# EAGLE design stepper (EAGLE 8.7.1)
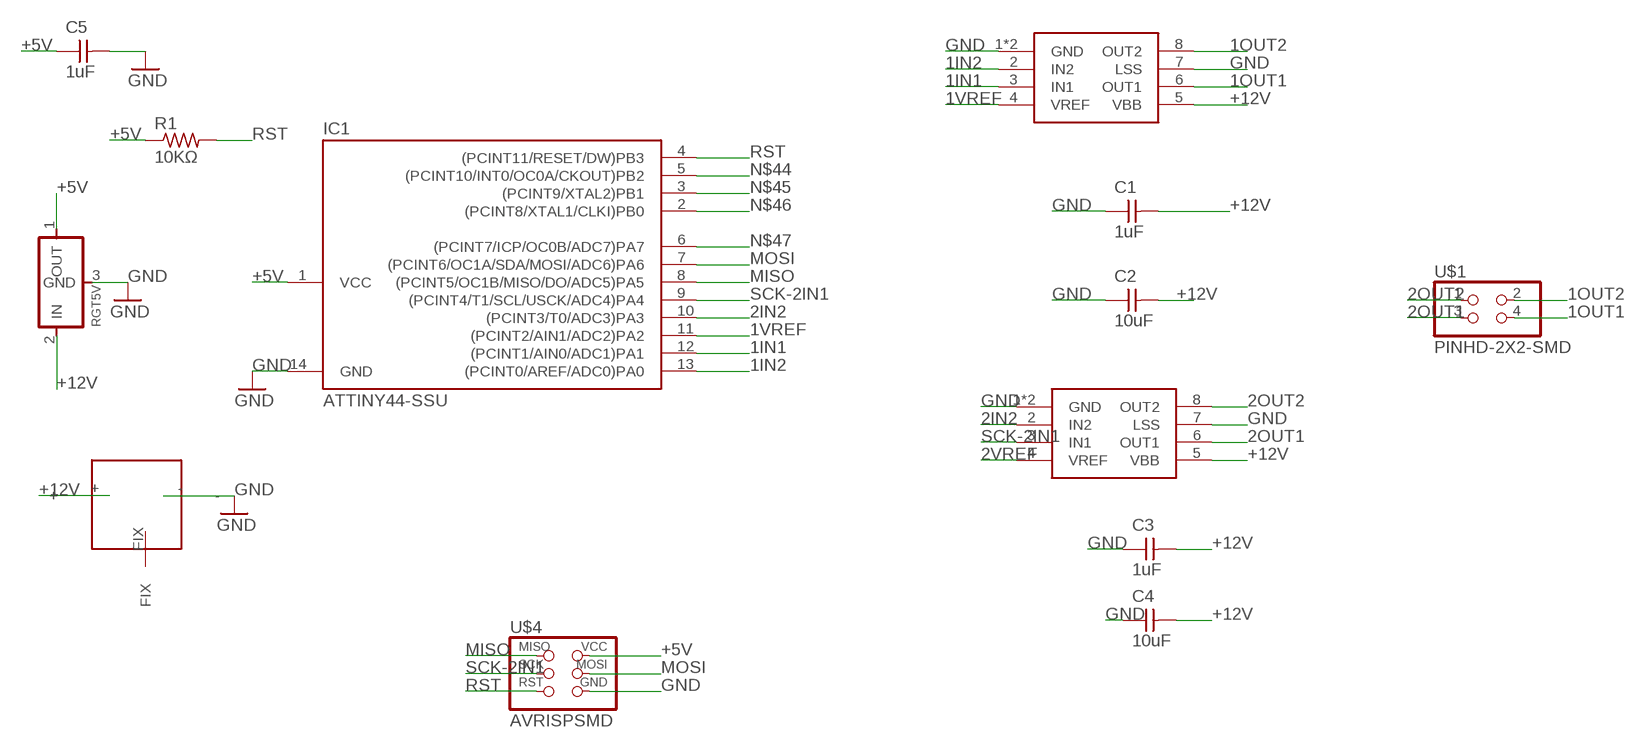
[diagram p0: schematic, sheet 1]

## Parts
C1  1uF  CAP-UNPOLARIZEDFAB  [C1206FAB]
C2  10uF  CAP-UNPOLARIZEDFAB  [C1206FAB]
C3  1uF  CAP-UNPOLARIZEDFAB  [C1206FAB]
C4  10uF  CAP-UNPOLARIZEDFAB  [C1206FAB]
C5  1uF  CAP-UNPOLARIZEDFAB  [C1206FAB]
DCJACK1  AKIZUKI_DCJACK  [AKIZUKI_DCJACK]
IC1  ATTINY44-SSU  [SOIC14]
R1  10KΩ  RES-US1206FAB  [R1206FAB]
RGT5V  REGULATORSOT23  [SOT23]
U$1  PINHD-2X2-SMD  [2X02SMD]
U$2  A4953-H-BRIDGE-MOTOR-DRIVER-PAD  [SOIC8_PAD]
U$3  A4953-H-BRIDGE-MOTOR-DRIVER-PAD  [SOIC8_PAD]
U$4  AVRISPSMD  [2X03SMD]

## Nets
1IN1: IC1.12((PCINT1/AIN0/ADC1)PA1) U$3.3(IN1)
1IN2: IC1.13((PCINT0/AREF/ADC0)PA0) U$3.2(IN2)
1OUT1: U$1.4 U$3.6(OUT1)
1OUT2: U$1.2 U$3.8(OUT2)
1VREF: IC1.11((PCINT2/AIN1/ADC2)PA2) U$3.4(VREF)
2IN2: IC1.10((PCINT3/T0/ADC3)PA3) U$2.2(IN2)
2OUT1: U$1.3 U$2.6(OUT1)
2OUT2: U$1.1 U$2.8(OUT2)
2VREF: U$2.4(VREF)
+5V: C5.1 IC1.1(VCC) R1.1 RGT5V.1(OUT) U$4.2(VCC)
+12V: C1.2 C2.2 C3.2 C4.2 DCJACK1.+ RGT5V.2(IN) U$2.5(VBB) U$3.5(VBB)
GND: C1.1 C2.1 C3.1 C4.1 C5.2 DCJACK1.- IC1.14(GND) RGT5V.3(GND) U$2.1(GND) U$2.7(LSS) U$2.GND U$3.1(GND) U$3.7(LSS) U$3.GND U$4.6(GND)
MISO: IC1.8((PCINT5/OC1B/MISO/DO/ADC5)PA5) U$4.1(MISO)
MOSI: IC1.7((PCINT6/OC1A/SDA/MOSI/ADC6)PA6) U$4.4(MOSI)
N$44: IC1.5((PCINT10/INT0/OC0A/CKOUT)PB2)
N$45: IC1.3((PCINT9/XTAL2)PB1)
N$46: IC1.2((PCINT8/XTAL1/CLKI)PB0)
N$47: IC1.6((PCINT7/ICP/OC0B/ADC7)PA7)
RST: IC1.4((PCINT11/RESET/DW)PB3) R1.2 U$4.5(RST)
SCK-2IN1: IC1.9((PCINT4/T1/SCL/USCK/ADC4)PA4) U$2.3(IN1) U$4.3(SCK)
Unconnected: DCJACK1.FIX

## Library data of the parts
C1-C5 = fab:CAP-UNPOLARIZED
DCJACK1 = doyo:AKIZUKI_DCJACK
IC1 = fab:ATTINY44
R1 = HelloKamakura:RES-US: Resistor (US Symbol)
RGT5V = fab:REGULATOR
U$1 = fab:PINHD-2X2-SMD
U$2 U$3 = fab:A4953-H-BRIDGE-MOTOR-DRIVER-PAD
U$4 = HelloKamakura:AVRISP

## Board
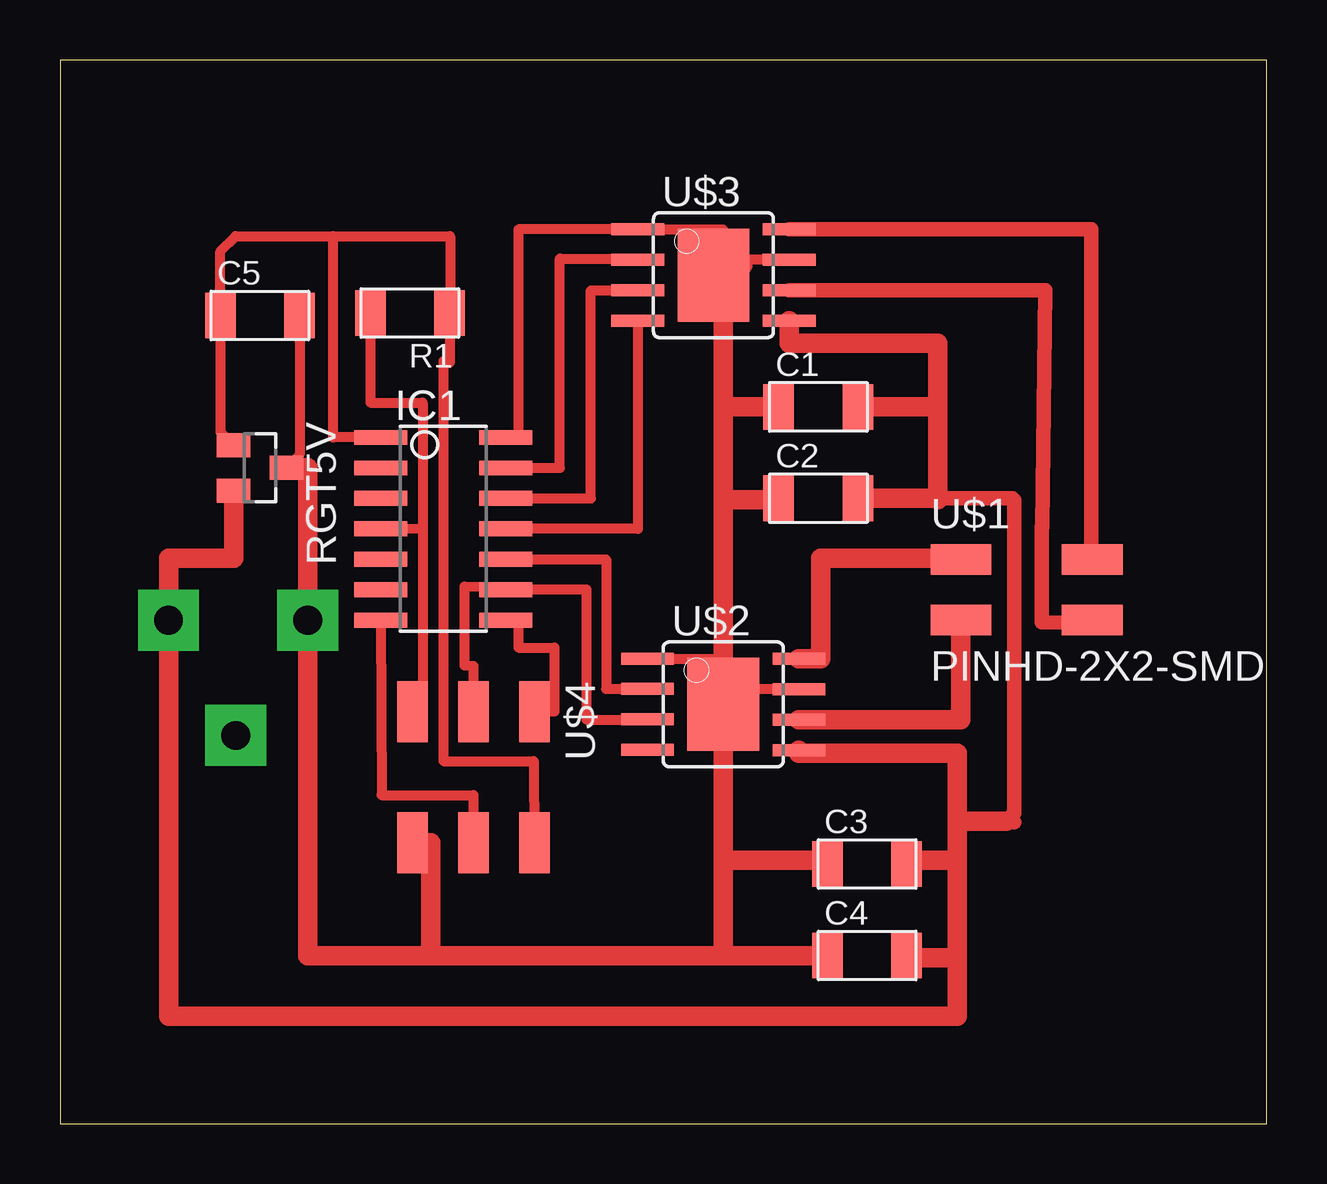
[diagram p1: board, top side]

Size 50.27 x 44.32 mm. Coordinates in mm from the lower left corner, seen from the top.
Outline: 0,0 50.27,0 50.27,44.32 0,44.32 0,0
Copper layers (1*16): Top 0.035mm / dielectric 1.5mm / Bottom 0.035mm
Design rules "default *": minimum track width 6mil, minimum drill 0.35mm, track to track 0.4mm, track to pad 0.4mm, pad to pad 0.4mm, via to via 0.4mm, smd to smd 0.4mm, copper to edge 40mil, drill to drill 6mil, minimum pad ring 10mil, minimum via ring 8mil, stop-mask expansion 4mil, vias tented up to drill 0mil, thermal gap 10mil

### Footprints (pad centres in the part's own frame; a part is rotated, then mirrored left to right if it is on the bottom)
C1206FAB = smd 1.27 x 1.905: 1 -1.651,0; 2 1.651,0
AKIZUKI_DCJACK = drill 1.2 pad 2.54 square: + 0,0; - 0,5.8; FIX 4.8,2.8
SOIC14 = smd 0.61 x 2.21: 1 -3.81,-2.603; 2 -2.54,-2.603; 3 -1.27,-2.603; 4 0,-2.603; 5 1.27,-2.603; 6 2.54,-2.603; 7 3.81,-2.603; 8 3.81,2.603; 9 2.54,2.603; 10 1.27,2.603; 11 0,2.603; 12 -1.27,2.603; 13 -2.54,2.603; 14 -3.81,2.603
R1206FAB = smd 1.27 x 1.905: 1 -1.651,0; 2 1.651,0
SOT23 = smd 1 x 1.4: 1 -0.95,-1.1; 2 0.95,-1.1; 3 0,1.1
2X02SMD = smd 2.54 x 1.27: 1 -2.54,1.27; 2 2.92,1.27; 3 -2.54,-1.27; 4 2.92,-1.27
SOIC8_PAD = smd 0.5 x 2.2: 1 -1.905,-3.154; 2 -0.645,-3.154; 3 0.625,-3.154; 4 1.895,-3.154; 5 1.905,3.154; 6 0.635,3.154; 7 -0.635,3.154; 8 -1.905,3.154 | smd 3.886 x 2.997: GND 0,0
2X03SMD = smd 2.54 x 1.27: 1 -2.54,2.54; 2 2.92,2.54; 3 -2.54,0; 4 2.92,0; 5 -2.54,-2.54; 6 2.92,-2.54

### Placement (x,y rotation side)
C1  31.6,29.87 0 top
C2  31.6,26.06 0 top
C3  33.63,10.82 0 top
C4  33.63,7.01 0 top
C5  8.33,33.68 0 top
DCJACK1  4.52,20.98 270 top
IC1  15.98,24.79 270 top
R1  14.58,33.78 180 top
RGT5V  8.33,27.33 270 top
U$1  40.08,22.25 0 top
U$2  27.64,17.48 270 top
U$3  27.23,35.36 270 top
U$4  17.22,14.63 270 top

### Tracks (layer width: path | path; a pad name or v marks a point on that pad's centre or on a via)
1IN1
  Top 0.406: IC1.12 22.12,26.06 22.12,34.72 U$3.3
1IN2
  Top 0.406: IC1.13 20.83,27.33 20.83,36.04 24.07,36.04 U$3.2
1OUT1
  Top 0.61: U$3.6 41.05,34.72 40.92,24.86 40.9,24.89 40.9,20.9 43.51,20.88 43.51,20.85 43,20.85 U$1.4
1OUT2
  Top 0.61: U$3.8 42.98,37.26 42.98,23.52 43.08,23.52
  Top 0.813: 43.08,23.52 U$1.2
1VREF
  Top 0.406: U$3.4 24.07,24.79 IC1.11
2IN2
  Top 0.406: IC1.10 22.76,23.52 22.76,18.12 U$2.2
2OUT1
  Top 0.813: U$2.6 37.54,16.84 U$1.3
2OUT2
  Top 0.813: U$2.8 31.7,19.38 31.7,23.57 37.54,23.57 U$1.1
+5V
  Top 0.406: 11.38,36.98 7.32,36.98 6.68,36.35 C5.1 6.68,28.83 RGT5V.1 | 11.38,36.98 16.26,36.98 16.26,33.81 R1.1 16.23,31.7 15.98,31.77 15.98,15.11 19.74,15.11 | 19.74,15.11 19.74,15.06 | 19.74,15.11 U$4.2 | IC1.1 11.38,28.6 11.38,36.98
+12V
  Top 0.61: 39.75,12.57 39.42,12.6 39.75,12.93 39.75,25.98 39.67,26.06 36.17,26.06
  Top 0.813: RGT5V.2 7.23,23.57 4.52,23.57 DCJACK1.+ 4.52,4.47 37.39,4.47 37.39,6.91 | 36.58,26.06 36.58,29.87 | 36.58,29.87 36.58,32.51 30.38,32.51 U$3.5 | C2.2 36.17,26.06 36.58,26.06 | 36.58,26.06 36.58,26.01 | C1.2 36.58,29.87 | 37.39,6.91 37.39,10.97 | 37.39,10.97 37.39,12.6 | 37.39,12.6 39.42,12.6 | C3.2 35.28,10.97 37.39,10.97 | C4.2 35.28,6.91 37.39,6.91 | U$2.5 30.79,15.44 37.39,15.44 37.39,12.6
GND
  Top 0.406: C5.2 9.98,27.88 RGT5V.3 | U$2.7 28.45,18.11 28.45,17.88 27.64,17.88 27.64,18.29 | U$2.1 27.64,19.38 27.64,18.69 | U$3.7 27.64,35.99 | 27.64,35.99 27.64,35.76 | 27.64,35.99 27.64,37.26 U$3.1 19.1,37.26 19.1,28.6 IC1.14
  Top 0.813: RGT5V.3 10.32,27.33 DCJACK1.- 10.32,7.01 15.44,7.01 | 15.44,7.01 27.64,7.01 | 27.64,7.01 C4.1 | U$4.6 15.44,11.71 15.44,7.01 | C2.1 29.95,26.01 27.64,26.01 | 27.64,10.97 U$2.GND 27.64,18.29 27.64,18.69 27.64,26.01 | 27.64,10.97 27.64,7.01 | 27.64,26.01 27.64,29.87 | 27.64,29.87 27.64,35.76 28.45,35.76 U$3.GND | C1.1 27.64,29.87 | 27.64,10.97 31.98,10.97 C3.1
MISO
  Top 0.406: IC1.8 19.1,20.98 19.1,19.84 20.6,19.84 20.6,17.17 U$4.1
MOSI
  Top 0.406: IC1.7 13.4,13.69 17.22,13.69 U$4.4
RST
  Top 0.406: R1.2 12.93,30.05 15.11,30.05 15.11,24.82 | 15.11,24.82 15.11,17.2 U$4.5 | IC1.4 15.11,24.82
SCK-2IN1
  Top 0.406: U$2.3 21.95,16.84 21.95,22.25 IC1.9 18.47,22.36 17.88,22.36 | 18.61,22.35 17.88,22.36 | 17.88,22.36 16.85,22.38 16.85,19.1 17.22,19.07 U$4.3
